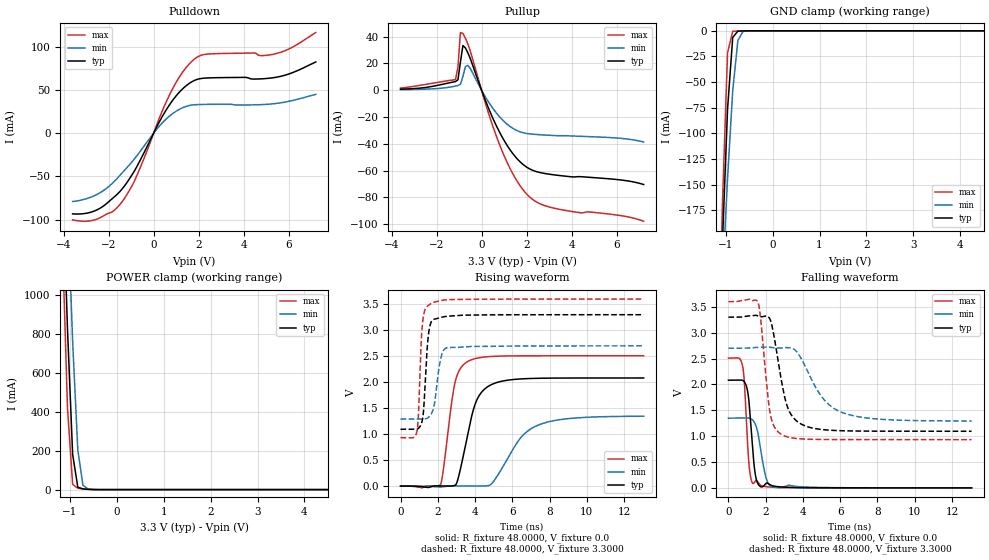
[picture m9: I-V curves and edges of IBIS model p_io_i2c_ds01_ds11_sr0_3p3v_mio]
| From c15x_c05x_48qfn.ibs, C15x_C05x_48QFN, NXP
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[Model] p_io_i2c_ds01_ds11_sr0_3p3v_mio
|   Model p_io_i2c_ds01_ds11_sr0_3p3v_mio
| This model was characterised for following simulation conditions:
| External (pad) voltage:
|   - Typ: 3.3V,   - Min: 2.7V,   - Max: 3.6V
| Library cells for typ/min/max conditions are connected as defined below:
|  pad - External Pad
|  ipp_do_lv - Core Input
|  ipp_obe_lv - Output Buffer Enable
|  IOGC - NC
|  REFH3V3 - REFH3V3
|  REFL3V3 - REFL3V3
|  ZI - NC
|  abut_ncal_vddio[1] - vddio
|  abut_ncal_vddio[2] - vddio
|  abut_ncal_vddio[3] - vssio
|  abut_ncal_vddio[4] - vddio
|  abut_ncal_vddio[5] - vddio
|  abut_ncal_vddio[6] - vssio
|  abut_pcal_vddio[1] - vssio
|  abut_pcal_vddio[2] - vssio
|  abut_pcal_vddio[3] - vddio
|  abut_pcal_vddio[4] - vssio
|  abut_pcal_vddio[5] - vssio
|  abut_pcal_vddio[6] - vddio
|  ipp_do_1p8v - ipp_do_1p8v
|  ipp_dse_lv[0] - vdd_lv
|  ipp_dse_lv[1] - vdd_lv
|  ipp_eftd_lv - NC
|  ipp_ina_mux_vddio - NC
|  ipp_ina_mux_vddio[0] - NC
|  ipp_ina_mux_vddio[1] - NC
|  ipp_ina_r0_vddio - NC
|  ipp_ina_r0a_vddio - NC
|  ipp_ina_r0b_vddio - NC
|  ipp_ina_r0c_vddio - NC
|  ipp_ina_r0d_vddio - NC
|  ipp_ina_r0e_vddio - NC
|  ipp_ina_r0f_vddio - NC
|  ipp_ina_r300_vddio - NC
|  ipp_ina_r300a_vddio - NC
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Model_type I/O
Polarity   Non-Inverting
Enable   Active-High
Vinl =   0.9900V
Vinh =   2.3100V
Vmeas =  1.6500V
Cref =   30.0000pF
Rref =   1.0000M
Vref =   3.3000V
C_comp   1.4149pF   1.3702pF   1.4746pF
|C_comp_pullup   0.5852pF   0.6306pF   0.5566pF
|C_comp_pulldown   0.7311pF   0.7417pF   0.7173pF
[Model Spec]
| variable   typ   min   max
Vinh   2.3100V   1.8900V   2.5200V
Vinl   0.9900V   0.8100V   1.0800V
[Temperature Range]   25.0000   0.1250k   -40.0000
[Voltage Range]   3.3000V   2.7000V   3.6000V
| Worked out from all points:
|   slope of the pulldown table from 0 to 0.495 V, typ, clamps not added: 20.5 ohm
|   slope of the pullup table from 0 to 0.495 V, typ, clamps not added: 23.9 ohm
|   GND clamp passes 1 mA (typ) near -0.75 V on its own axis
|   POWER clamp passes 1 mA (typ) near -0.57 V on its own axis
|   rising waveform, R_fixture 48.0000, V_fixture 0.0: 20-80 % time 834ps typ, 1.56ns min, 565ps max; typ from 0 V to 2.08 V
|   rising waveform, R_fixture 48.0000, V_fixture 3.3000: 20-80 % time 228ps typ, 321ps min, 190ps max; typ from 1.09 V to 3.3 V
|   falling waveform, R_fixture 48.0000, V_fixture 0.0: 20-80 % time 282ps typ, 395ps min, 231ps max; typ from 2.08 V to 0 V
|   falling waveform, R_fixture 48.0000, V_fixture 3.3000: 20-80 % time 715ps typ, 1.48ns min, 442ps max; typ from 3.3 V to 1.09 V
[Pulldown]
|Voltage   I(typ)   I(min)   I(max)
-3.6V     -93.31mA   -79.05mA   -100.2mA
-2.5V     -88.48mA   -70.63mA   -99.19mA
-1.84V    -75.78mA   -58.1mA    -91mA
-1.4V     -64.51mA   -45.95mA   -79.27mA
-850mV    -43.59mA   -29.61mA   -55.29mA
140mV     7.403mA    4.641mA    9.826mA
800mV     36.32mA    21.74mA    49.15mA
1.35V     52.7mA     30.01mA    72.7mA
1.79V     60.61mA    32.73mA    85.13mA
2.45V     63.81mA    33.25mA    91.42mA
5.42V     64.46mA    34.22mA    91.77mA
7.2V      82.23mA    44.78mA    116.2mA
[Pullup]
|Voltage   I(typ)   I(min)   I(max)
-3.6V     785.4uA    423.3uA    1.608mA
-1.16V    6.455mA    3.098mA    7.926mA
-1.05V    7.777mA    3.482mA    16.99mA
-940mV    20.9mA     4.372mA    43.05mA
-830mV    33.33mA    10.25mA    42.41mA
-720mV    31.61mA    17.65mA    38.91mA
-610mV    27.98mA    18.58mA    34.56mA
820mV     -32.01mA   -20.24mA   -41.48mA
1.48V     -49.28mA   -29.34mA   -65.19mA
2.03V     -57.72mA   -32.35mA   -77.98mA
3.24V     -63.24mA   -33.85mA   -88.14mA
7.2V      -70.41mA   -38.61mA   -97.87mA
[GND_clamp]
|Voltage   I(typ)   I(min)   I(max)
-3.6V     -4.327A    -3.181A    -5.901A
-1.18V    -358.9mA   -350.6mA   -379.3mA
-1.07V    -208.2mA   -244.2mA   -170.8mA
-960mV    -76.59mA   -144.3mA   -21.58mA
-850mV    -6.561mA   -58.74mA   -508.1uA
-740mV    -273.3uA   -9.382mA   -183.5uA
-630mV    -73.8uA    -593.1uA   -76.7uA
-410mV    -3.432uA   -9.016uA   -2.096uA
7.2V      0A         0A         0A
[POWER_clamp]
|Voltage   I(typ)   I(min)   I(max)
-3.6V     20.44A     18.76A     22.48A
-1.16V    1.647A     2.216A     1.289A
-1.05V    823.6mA    1.482A     419.2mA
-940mV    180.4mA    758.9mA    26.72mA
-830mV    12.56mA    202.9mA    6.794mA
-720mV    3.422mA    22.23mA    3.58mA
-610mV    1.373mA    2.923mA    1.344mA
7.2V      0A         0A         0A
[Ramp]
| variable   typ   min   max
dV/dt_r  1.2489/0.8345n   0.8072/1.5638n   1.5056/0.5650n
dV/dt_f  1.3235/0.7146n   0.8448/1.4834n   1.6008/0.4417n
R_load = 48.0000
[Rising Waveform]
R_fixture= 48.0000
V_fixture= 0.0
V_fixture_min= 0.0
V_fixture_max= 0.0
|time   V(typ)   V(min)   V(max)
0s        1.113nV    81.31nV    3.704nV
2.149ns   3.461mV    -17.78mV   31.05mV
2.931ns   15.25mV    1.881mV    2.005V
3.139ns   212.7mV    1.921mV    2.219V
3.603ns   997.4mV    1.205mV    2.398V
4.176ns   1.716V     -1.357mV   2.468V
5.187ns   1.996V     191.1mV    2.501V
6.423ns   2.063V     918.5mV    2.508V
7.46ns    2.076V     1.184V     2.509V
13.05ns   2.082V     1.345V     2.509V
[Rising Waveform]
R_fixture= 48.0000
V_fixture= 3.3000
V_fixture_min= 2.7000
V_fixture_max= 3.6000
|time   V(typ)   V(min)   V(max)
0s        1.094V     1.29V      932mV
888.4ps   1.097V     1.29V      1.067V
963.5ps   1.112V     1.29V      1.385V
1.143ns   1.228V     1.29V      2.977V
1.245ns   1.495V     1.29V      3.304V
1.458ns   2.772V     1.312V     3.469V
1.629ns   3.145V     1.378V     3.513V
2.17ns    3.248V     2.476V     3.571V
2.469ns   3.268V     2.662V     3.587V
13.05ns   3.3V       2.7V       3.6V
[Falling Waveform]
R_fixture= 48.0000
V_fixture= 0.0
V_fixture_min= 0.0
V_fixture_max= 0.0
|time   V(typ)   V(min)   V(max)
0s        2.082V     1.348V     2.509V
764ps     2.078V     1.348V     2.346V
853.4ps   2.05V      1.348V     2.05V
1.103ns   1.66V      1.349V     454.4mV
1.316ns   671.8mV    1.304V     83.49mV
1.443ns   256.9mV    1.23V      131.1mV
1.588ns   74.42mV    1.048V     110.6mV
2.004ns   81.84mV    214.6mV    22.64mV
2.337ns   42.85mV    20.54mV    13.07mV
13.05ns   2.124uV    26.59uV    355.7nV
[Falling Waveform]
R_fixture= 48.0000
V_fixture= 3.3000
V_fixture_min= 2.7000
V_fixture_max= 3.6000
|time   V(typ)   V(min)   V(max)
0s        3.3V       2.7V       3.6V
1.592ns   3.323V     2.717V     3.583V
1.728ns   3.309V     2.719V     3.269V
2.225ns   3.264V     2.719V     1.465V
2.878ns   2.006V     2.704V     1.026V
3.185ns   1.547V     2.711V     983mV
3.667ns   1.291V     2.631V     953.6mV
4.974ns   1.129V     1.778V     935.5mV
6.062ns   1.105V     1.463V     933.2mV
13.05ns   1.094V     1.292V     932.1mV
